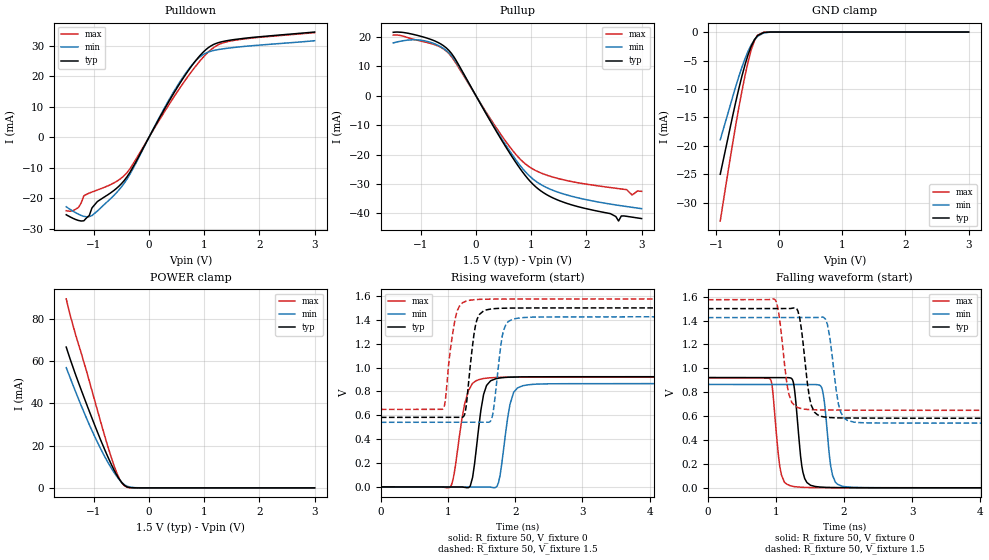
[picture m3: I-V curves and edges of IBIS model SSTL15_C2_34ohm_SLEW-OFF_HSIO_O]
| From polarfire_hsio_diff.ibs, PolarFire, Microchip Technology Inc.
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|   Model SSTL15_C2_34ohm_SLEW-OFF_HSIO_O
[Model]   SSTL15_C2_34ohm_SLEW-OFF_HSIO_O
Model_type   Output
Polarity   Non-Inverting
Enable   Active-High
Vmeas =   0.75
Cref =   5p
Rref =   50
Vref =   0.75
|   typ   min   max
C_comp_pullup   1.335e-12   1.335e-12   1.380e-12
C_comp_pulldown  1.335e-12   1.335e-12   1.380e-12
[Temperature Range]  25C   100C   -40C
[Voltage Range]  1.5   1.425   1.575
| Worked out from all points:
|   slope of the pulldown table from 0 to 0.225 V, typ, clamps not added: 30.1 ohm
|   slope of the pullup table from 0 to 0.225 V, typ, clamps not added: 30.2 ohm
|   GND clamp passes 1 mA (typ) near -0.37 V on its own axis
|   POWER clamp passes 1 mA (typ) near -0.43 V on its own axis
|   rising waveform, R_fixture 50, V_fixture 0: 20-80 % time 126ps typ, 128ps min, 156ps max; typ from 0 V to 0.923 V
|   rising waveform, R_fixture 50, V_fixture 1.5: 20-80 % time 110ps typ, 110ps min, 122ps max; typ from 0.582 V to 1.5 V
|   falling waveform, R_fixture 50, V_fixture 0: 20-80 % time 91.1ps typ, 91.1ps min, 90.3ps max; typ from 0.923 V to 0 V
|   falling waveform, R_fixture 50, V_fixture 1.5: 20-80 % time 112ps typ, 119ps min, 114ps max; typ from 1.5 V to 0.582 V
[GND Clamp]
| Voltage   I(typ)   I(min)   I(max)
-935.2mV  -24.96mA   -18.92mA   -33.17mA
-738.3mV  -14.72mA   -11.38mA   -19.54mA
-639.8mV  -9.903mA   -7.788mA   -13.22mA
-590.6mV  -7.7mA     -6.143mA   -10.29mA
-541.4mV  -5.692mA   -4.645mA   -7.577mA
-492.2mV  -3.93mA    -3.33mA    -5.153mA
-443mV    -2.467mA   -2.229mA   -3.103mA
-393.7mV  -1.355mA   -1.366mA   -1.54mA
-344.5mV  -621.9uA   -750.5uA   -567.2uA
-246.1mV  -72.57uA   -154.2uA   -30.93uA
-147.7mV  -5.325uA   -20.63uA   -1.146uA
3V        0A         0A         0A
[POWER Clamp]
| Voltage   I(typ)   I(min)   I(max)
-1.5V     66.64mA    56.9mA     89.46mA
-1.427V   60.81mA    51.96mA    81.57mA
-1.329V   53.43mA    45.4mA     72.34mA
-1.083V   36.31mA    29.95mA    50.59mA
-885.9mV  23.26mA    18.98mA    32.15mA
-738.3mV  14.22mA    11.74mA    18.91mA
-590.6mV  6.331mA    5.649mA    7.47mA
-492.2mV  2.418mA    2.54mA     2.302mA
-443mV    1.134mA    1.422mA    896.4uA
-344.5mV  93.53uA    323uA      39.71uA
-246.1mV  3.484uA    76.21uA    1.361uA
3V        0A         0A         0A
[Pullup]
| Voltage   I(typ)   I(min)   I(max)
-1.5V     21.63mA    18.02mA    20.68mA
-935.2mV  19.92mA    18.75mA    18.37mA
-492.2mV  15.48mA    14.66mA    14.41mA
609.4mV   -19.45mA   -18.72mA   -17.29mA
890.6mV   -27.08mA   -25.75mA   -23.1mA
1.172V    -32.3mA    -30.13mA   -26.2mA
1.648V    -36.59mA   -33.73mA   -28.83mA
2.435V    -40.08mA   -36.83mA   -31.2mA
2.583V    -42.58mA   -37.25mA   -31.56mA
2.632V    -40.87mA   -37.39mA   -31.68mA
2.829V    -41.27mA   -37.93mA   -33.74mA
3V        -41.75mA   -38.38mA   -32.49mA
[Pulldown]
| Voltage   I(typ)   I(min)   I(max)
-1.5V     -25.45mA   -22.84mA   -24.12mA
-1.28V    -27.33mA   -25.27mA   -23.09mA
-1.181V   -27.44mA   -25.97mA   -19.25mA
-1.083V   -25.71mA   -26.08mA   -18.35mA
-935.2mV  -21.11mA   -24.24mA   -17.32mA
-590.6mV  -16.81mA   -18.24mA   -14.53mA
-344.5mV  -11.51mA   -12.11mA   -10.34mA
562.5mV   17.79mA    18.29mA    16.26mA
843.8mV   25.11mA    25.06mA    23.29mA
1.078V    29.46mA    28mA       28.04mA
1.5V      31.96mA    29.4mA     31.68mA
3V        34.55mA    31.69mA    34.33mA
[Ramp]
dV/dt_r   0.554086/0.1257n  0.51933/0.127747n  0.551931/0.156382n
dV/dt_f   0.550552/0.11238n  0.53034/0.11946n  0.55563/0.114456n
R_load = 50
[Rising Waveform]
R_fixture = 50
V_fixture = 0
V_fixture_min = 0
V_fixture_max = 0
| Time   V(typ)   V(min)   V(max)
0s        1.606uV    1.724uV    2.5uV
1.028ns   -809.7uV   -623.3uV   -4.196mV
1.305ns   -6.307mV   -791.7uV   807.4mV
1.366ns   79.83mV    -828.8uV   867.6mV
1.518ns   736.5mV    -921.2uV   907mV
1.574ns   850mV      -955.3uV   911mV
1.752ns   910.5mV    36.92mV    917.3mV
1.923ns   919.6mV    693.1mV    918.3mV
2.112ns   921.8mV    847.4mV    918.7mV
10ns      923.5mV    865.6mV    919.9mV
[Rising Waveform]
R_fixture = 50
V_fixture = 1.5
V_fixture_min = 1.425
V_fixture_max = 1.575
| Time   V(typ)   V(min)   V(max)
0s        582.4mV    541.1mV    648.9mV
927ps     582.9mV    541.5mV    655.1mV
1.122ns   583mV      541.6mV    1.446V
1.248ns   608.4mV    541.7mV    1.551V
1.326ns   985.1mV    541.7mV    1.564V
1.435ns   1.408V     541.8mV    1.57V
1.648ns   1.491V     567.8mV    1.573V
1.825ns   1.497V     1.309V     1.574V
1.975ns   1.498V     1.407V     1.574V
10ns      1.5V       1.425V     1.575V
[Falling Waveform]
R_fixture = 50
V_fixture = 0
V_fixture_min = 0
V_fixture_max = 0
| Time   V(typ)   V(min)   V(max)
0s        923.5mV    865.6mV    919.9mV
918ps     922.7mV    865.1mV    908.7mV
1.081ns   922.6mV    865mV      107.1mV
1.278ns   796.4mV    864.9mV    9.661mV
1.363ns   258.9mV    864.8mV    5.426mV
1.423ns   76.42mV    864.8mV    3.85mV
1.674ns   5.918mV    833.7mV    1.636mV
1.832ns   2.659mV    102.1mV    1.21mV
1.969ns   1.693mV    14mV       972.4uV
10ns      2.565uV    2.947uV    3.271uV
[Falling Waveform]
R_fixture = 50
V_fixture = 1.5
V_fixture_min = 1.425
V_fixture_max = 1.575
| Time   V(typ)   V(min)   V(max)
0s        1.5V       1.425V     1.575V
997ps     1.501V     1.425V     1.568V
1.188ns   1.501V     1.426V     787.1mV
1.322ns   1.481V     1.426V     671.7mV
1.388ns   1.261V     1.426V     661.4mV
1.566ns   633.2mV    1.426V     653.1mV
1.754ns   590.3mV    1.372V     651.6mV
1.918ns   585.7mV    699.7mV    650.8mV
2.143ns   584.5mV    550.2mV    650.1mV
10ns      582.4mV    541.1mV    648.9mV
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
